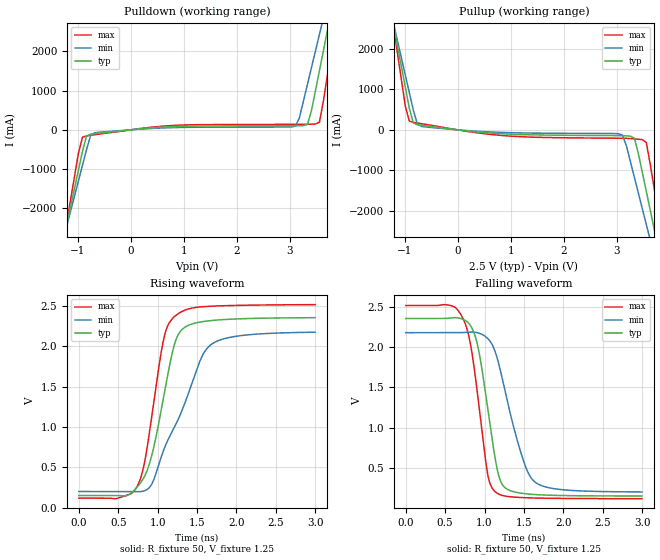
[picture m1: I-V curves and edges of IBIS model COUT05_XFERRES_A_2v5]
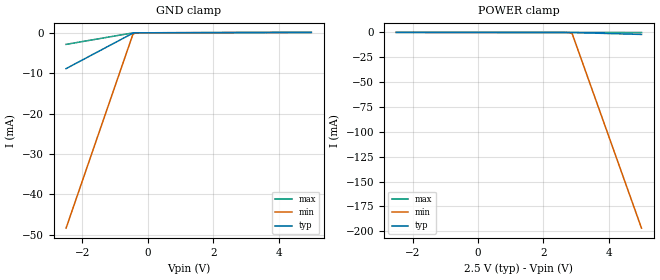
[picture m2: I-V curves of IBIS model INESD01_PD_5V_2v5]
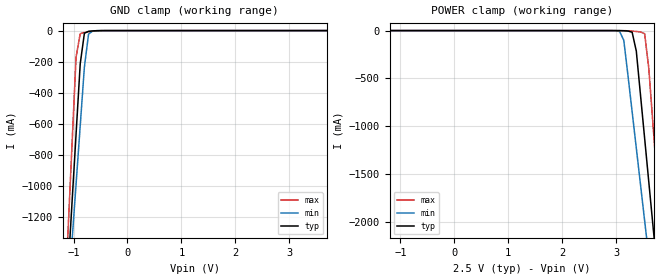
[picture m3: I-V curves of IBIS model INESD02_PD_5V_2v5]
|   This file is an IBIS representation of the   |
|   Integrated Device Technology, Inc.   |
|   ICS87002-02   |
|   1:2, DIFFERENTIAL-TO-LVCMOS/LVTTL ZERO DELAY CLOCK GENERATOR   |
[IBIS Ver]   4.1
[File name]   87002_02.ibs
[File Rev]   1.0
[Date]   16 Jun 2009 | Last modified
[Source]   Originated at Integrated Devices Technology, Inc.
[Disclaimer]
IDT hereby grants the user of this IBIS model a non-exclusive,
nontransferable license to use this IBIS model under the following terms.
Before using this IBIS model, the user should read this license.
If the user does not accept these terms,  the IBIS model should be
returned to IDT within 30 days.
   The user is granted this license only to use the IBIS model and
is not granted rights to sell, load, rent, lease or license the IBIS
model in whole or in part, or in modified form to anyone other than
user. User may modify the IBIS model to suit its specific
applications but rights to derivative works and such modifications
shall belong to IDT.
   This IBIS model is provided on an "AS IS" basis and IDT makes
absolutely no warranty with respect to the information contained
herein. IDT DISCLAIMS AND CUSTOMER WAIVES ALL WARRANTIES, EXPRESS
OR IMPLIED, INCLUDING WARRANTIES OF MERCHANTABILITY OR FITNESS FOR
A PARTICULAR PURPOSE. The entire risk as to quality and performance
is with the Customer. ACCORDINGLY, IN NO EVENT SHALL THE COMPANY BE
LIABLE FOR ANY DAMAGES, WHETHER IN CONTRACT OR TORT,INCLUDING ANY
LOST PROFITS OR OTHER INCIDENTAL, CONSEQUENTIAL, EXEMPLARY, OR
PUNITIVE DAMAGES ARISING OUT OF THE USE OR APPLICATION OF THE IBIS
model provided in this package. Further, IDT reserves the right to
make changes without notice to any product herein to improve
reliability, function, or design. IDT does not convey any license
under patent rights or any other intellectual property rights,
including those of third parties.
   IDT is not obligated to provide maintenance or support
for the licensed IBIS model.
[Copyright]   Copyright 2005 by Integrated Device Technology, Inc.
[Component]   ICS87002G-02
[Manufacturer] Integrated Devices Technology, Inc.
[Package]
|TSSOP 20 Lead
|   typ   min   max
R_pkg   51.85m   41.1m   62.6m
L_pkg   1.568nH   0.734nH   2.401nH
C_pkg   0.221pF   0.068pF   0.373pF
[Pin] signal_name   model_name   R_pin   L_pin   C_pin
1  GND   GND   62.6m   2.401n   0.373p
2  Q0   COUT05_XFERRES_A   57.23m   1.985n   0.297p
3  VDDO   POWER   51.85m   1.568n   0.221p
4  SEL0   INESD01_PD_5V   46.78m   1.151n   0.145p
5  SEL1   INESD01_PD_5V   41.1m   0.734n   0.068p
6  SEL2   INESD01_PD_5V   41.1m   0.734n   0.068p
7  SEL3   INESD01_PD_5V   46.78m   1.151n   0.145p
8  VDD   POWER   51.85m   1.568n   0.221p
9  CLK   INESD02_PD_5V   57.23m   1.985n   0.297p
10 nCLK   INESD02_PMID_5V   62.6m   2.401n   0.373p
11 GND   GND   62.6m   2.401n   0.373p
12 VDDA   POWER   57.23m   1.985n   0.297p
13 PLL_SEL   INESD01_PU_5V   51.85m   1.568n   0.221p
14 FB_IN   INESD02_PD_5V   46.78m   1.151n   0.145p
15 MR   INESD01_PD_5V   41.1m   0.734n   0.068p
16 NC   NC   41.1m   0.734n   0.068p
17 VDDO   POWER   46.78m   1.151n   0.145p
18 GND   GND   51.85m   1.568n   0.221p
19 Q1   COUT05_XFERRES_A   57.23m   1.985n   0.297p
20 VDDO   POWER   62.6m   2.401n   0.373p
[Diff Pin]  inv_pin  vdiff tdelay_typ tdelay_min  tdelay_max
9   10   0.15   0   0   0
[Model Selector] COUT05_XFERRES_A
COUT05_XFERRES_A_2v5  Buffer selection for 2v5
COUT05_XFERRES_A_3v3  Buffer selection for 3v3
[Model Selector] INESD01_PD_5V
INESD01_PD_5V_2v5  Buffer selection for 2v5
INESD01_PD_5V_3v3  Buffer selection for 3v3
[Model Selector] INESD02_PD_5V
INESD02_PD_5V_2v5  Buffer selection for 2v5
INESD02_PD_5V_3v3  Buffer selection for 3v3
[Model Selector] INESD02_PMID_5V
INESD02_PMID_5V_2v5  Buffer selection for 2v5
INESD02_PMID_5V_3v3  Buffer selection for 3v3
[Model Selector] INESD01_PU_5V
INESD01_PU_5V_2v5  Buffer selection for 2v5
INESD01_PU_5V_3v3  Buffer selection for 3v3
| Models and submodels in the file (10): COUT05_XFERRES_A_2v5 (Output), INESD01_PD_5V_2v5 (Input), INESD02_PD_5V_2v5 (Input), INESD02_PMID_5V_2v5 (Input), INESD01_PU_5V_2v5 (Input), COUT05_XFERRES_A_3v3 (Output), INESD01_PD_5V_3v3 (Input), INESD02_PD_5V_3v3 (Input), INESD02_PMID_5V_3v3 (Input), INESD01_PU_5V_3v3 (Input)
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[Model] COUT05_XFERRES_A_2v5
Model_type  Output
Polarity   Non-Inverting
Vmeas = 1.25
Rref = 50
Cref = 0
Vref = 1.25
|Variable  typ   min   max
C_comp   2p   1.5p   2.5p
[Voltage Range]   2.5   2.375   2.625
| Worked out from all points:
|   slope of the pulldown table from 0 to 0.375 V, typ, clamps not added: 7.84 ohm
|   slope of the pullup table from 0 to 0.375 V, typ, clamps not added: 7.17 ohm
|   rising waveform, R_fixture 50, V_fixture 1.25: 20-80 % time 274ps typ, 488ps min, 225ps max; typ from 0.154 V to 2.35 V
|   falling waveform, R_fixture 50, V_fixture 1.25: 20-80 % time 205ps typ, 309ps min, 191ps max; typ from 2.35 V to 0.154 V
| Open source, no load
|  Voltage   I(typ)   I(min)   I(max)
[Pullup]
-2.5V     11.44A     9.986A     13.84A
-1.212V   2.607A     2.64A      2.573A
-909.1mV  526mA      911.1mA    212mA
-833.3mV  167.1mA    478.9mA    184.4mA
-681.8mV  112.7mA    84.76mA    151.8mA
3.106V    -144.5mA   -124.8mA   -207.2mA
3.333V    -201.9mA   -1.16A     -222.3mA
3.485V    -1.051A    -1.943A    -242.2mA
3.561V    -1.521A    -2.334A    -315mA
3.712V    -2.464A    -3.118A    -1.472A
3.864V    -3.407A    -3.903A    -2.677A
5V        -10.49A    -9.798A    -11.71A
[Pulldown]
-2.5V     -10.49A    -9.183A    -12.66A
-1.288V   -2.917A    -2.872A    -3.01A
-1.212V   -2.443A    -2.477A    -2.405A
-909.1mV  -543.8mA   -898.7mA   -186.9mA
-833.3mV  -160.7mA   -504.4mA   -155.1mA
-757.6mV  -109mA     -149.4mA   -139.6mA
3.106V    103.9mA    93.06mA    139.6mA
3.333V    137.9mA    1.155A     141.5mA
3.561V    1.512A     2.434A     197.9mA
3.712V    2.539A     3.288A     1.405A
3.864V    3.567A     4.143A     2.72A
5V        11.31A     10.58A     12.63A
[Ramp]
|   typ   min   max
dV/dt_r   1.762/0.433n   1.577/0.660n   1.919/0.360n
dV/dt_f   1.769/0.311n   1.585/0.457n   1.923/0.297n
R_load =   50.0000
[Rising Waveform]
R_fixture = 50
V_fixture = 1.25   | VCC_typ
V_fixture_max = 1.3125   | VCC_max
V_fixture_min = 1.1875   | VCC_min
C_fixture = 0.0p
| Time   typ   min   max
0s        154.1mV    203.2mV    121.3mV
477.4ps   154.3mV    203.2mV    116.6mV
740.9ps   259.7mV    200.8mV    269.6mV
821.5ps   368.8mV    208.9mV    507.2mV
905.2ps   578.3mV    264.4mV    996.6mV
1.079ns   1.39V      722.9mV    2.098V
1.228ns   2.067V     1.027V     2.379V
1.553ns   2.301V     1.854V     2.487V
1.693ns   2.318V     2.03V      2.495V
2.998ns   2.352V     2.173V     2.513V
[Falling Waveform]
R_fixture = 50
V_fixture = 1.25   | VCC_typ
V_fixture_max = 1.3125   | VCC_max
V_fixture_min = 1.1875   | VCC_min
C_fixture = 0.0p
| Time   typ   min   max
0s        2.355V     2.179V     2.515V
725.4ps   2.344V     2.181V     2.356V
818.4ps   2.271V     2.187V     2.053V
911.4ps   2.026V     2.178V     1.415V
1.039ns   1.249V     2.109V     432mV
1.141ns   587mV      1.926V     202.8mV
1.259ns   258.4mV    1.464V     154.1mV
1.479ns   187.7mV    638mV      135.2mV
1.624ns   173.7mV    341.8mV    130.1mV
2.998ns   154.5mV    205mV      121.5mV
[Model] INESD01_PD_5V_2v5
Model_type   Input
Polarity   Non-Inverting
Vinl = 0.8V
Vinh = 2.0V
|   typ   min   max
C_comp   2pF   1.5pF   2.5pF
|   typ   min   max
[Voltage range]  2.5V   2.375V   2.625V
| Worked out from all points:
|   GND clamp passes 1 mA (typ) near -0.67 V on its own axis
[GND_clamp]
|Voltage   I(typ)   I(min)   I(max)
-2.5V     -8.873mA   -48.37mA   -2.87mA
-454.5mV  -90.52uA   -342uA     -24.79uA
-378.8mV  -21.06uA   -68.59uA   -9.129uA
-227.3mV  -4.664uA   -6.183uA   -4.627uA
5V        98.01uA    94.31uA    101.7uA
[POWER_clamp]
|Voltage   I(typ)   I(min)   I(max)
-2.5V     97.98uA    91.95uA    104.2uA
2.652V    -2.989uA   -11.36uA   -539.2nA
2.879V    -21.06uA   -1.086mA   -5.176uA
5V        -1.966mA   -196.9mA   -55.09uA
[Model] INESD02_PD_5V_2v5
Model_type   Input
Polarity   Non-Inverting
Vinl = .87V
Vinh = 1.62V
|   typ   min   max
C_comp   2pF   1.5pF   2.5pF
|   typ   min   max
[Voltage range]   2.5V   2.375V   2.625V
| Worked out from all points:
|   GND clamp passes 1 mA (typ) near -0.59 V on its own axis
[GND_clamp]
|Voltage   I(typ)   I(min)   I(max)
-2.191V   -7.973A    -7.07A     -9.504A
-1.108V   -1.581A    -1.751A    -1.338A
-1.031V   -1.125A    -1.371A    -755.2mA
-953.6mV  -669.5mA   -992.5mA   -172.1mA
-876.3mV  -213.9mA   -613.7mA   -19.96mA
-799mV    -17.31mA   -235.3mA   -12.11mA
-721.6mV  -4.455mA   -23.01mA   -7.724mA
-644.3mV  -1.863mA   -2.522mA   -4.06mA
5V        97.41uA    121.8uA    75.48uA
[POWER_clamp]
|Voltage   I(typ)   I(min)   I(max)
-2.5V     97.41uA    118.8uA    77.37uA
2.835V    -9.233uA   -44.7uA    -3.208uA
3.067V    -617.5uA   -9.489mA   -116.3uA
3.144V    -1.863mA   -101.8mA   -642.8uA
3.299V    -17.31mA   -847.2mA   -5.362mA
3.376V    -213.9mA   -1.226A    -9.326mA
3.531V    -1.125A    -1.985A    -32.65mA
3.608V    -1.581A    -2.364A    -395.6mA
3.686V    -2.038A    -2.744A    -978.8mA
3.763V    -2.494A    -3.124A    -1.562A
3.84V     -2.95A     -3.503A    -2.145A
4.845V    -8.886A    -8.445A    -9.728A
